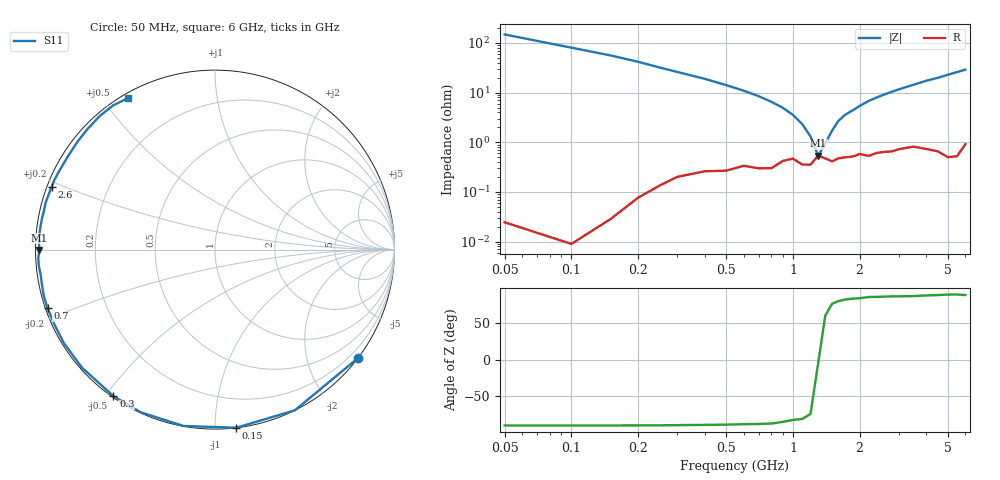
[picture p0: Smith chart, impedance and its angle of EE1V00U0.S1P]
! Infineon Technologies  Discrete & RF Semiconductors
! BBY55-02W
! Si Tuning Diode in SCD-80
! VR = 1 V
! S-Parameters:  June  2000
# GHz  S  MA  R  50
!  f  S11
! GHz  MAG  ANG
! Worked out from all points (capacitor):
!   34 points, 50 MHz to 6 GHz, reference 50 ohm
!   read as one part to ground: C = 19.6 pF near 50 MHz
!   lowest |Z| = 537 mohm at 1.3 GHz (marker M1)
!   series resonance near 1.305 GHz, so ESL is about 760 pH
!   S11 on the Smith chart (normalised r, x): 50 MHz: 0.00, -2.97; 150 MHz: 0.00, -1.13; 300 MHz: 0.00, -0.52; 700 MHz: 0.01, -0.17; 2.6 GHz: 0.01, +0.19; 6 GHz: 0.02, +0.58
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0.05  0.9999 -37.2
0.1  0.9999 -63.6
0.15  0.9995 -83.2
0.2  0.9982 -100.1
0.25  0.9962 -114.5
0.3  0.9937 -124.7
0.4  0.9909 -138.4
0.5  0.9901 -148.3
0.6  0.9872 -155.3
0.7  0.9884 -160.7
0.8  0.9882 -165.1
1  0.9815 -171.9
1.2  0.9859 -177.1
1.3  0.9788 -179.9
1.5  0.9836 176.2
1.6  0.9813 174.0
1.7  0.9804 172.2
1.9  0.9791 169.4
2.2  0.9792 164.5
2.4  0.9763 161.7
2.6  0.9754 159.0
3  0.9728 153.8
3.5  0.9702 147.8
4  0.9741 141.7
4.5  0.9775 136.6
5  0.9835 130.7
5.5  0.9836 125.1
6  0.9729 119.7
